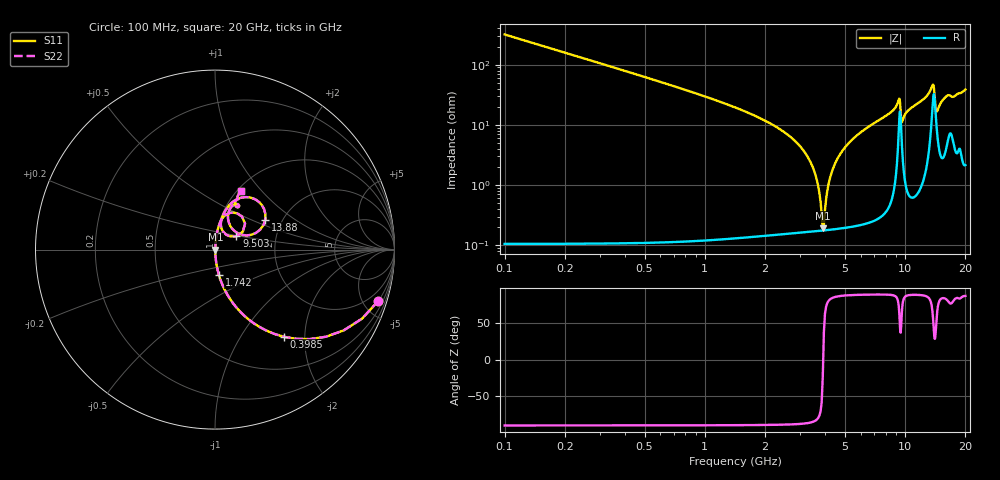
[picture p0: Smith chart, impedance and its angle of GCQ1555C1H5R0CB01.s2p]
!Murata Part Number: GCQ1555C1H5R0CB01
!These Parameters are Measured in Series Mode Connection
!Data Generated on Jan 08, 2026
!  o--ll--o
!Port1  Port2
!  o------o
!Operation Temp=25[degC], DC Bias Voltage=0[V]
!Freq. Start=100[MHz] Stop=20[GHz] 401[Steps]
# Hz S RI R 50
!Freq.(Hz) S11(Real) S11(Imag) S21(Real) S21(Imag) S12(Real) S12(Imag) S22(Real) S22(Imag)
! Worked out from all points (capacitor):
!   401 points, 100 MHz to 20 GHz, reference 50 ohm
!   read as one part in series: C = 5 pF near 199.5 MHz
!   lowest |Z| = 190 mohm at 3.881 GHz (marker M1)
!   series resonance near 3.898 GHz, so ESL is about 330 pH
!   S11 on the Smith chart (normalised r, x): 100 MHz: 1.00, -6.36; 398.5 MHz: 1.00, -1.58; 1.742 GHz: 1.00, -0.29; 9.503 GHz: 1.25, +0.19; 13.88 GHz: 1.64, +0.61; 20 GHz: 1.04, +0.77
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1e8  0.91 -0.286  0.09 0.286  0.09 0.286  0.91 -0.286
3.985e8  0.3847 -0.4858  0.6153 0.4858  0.6153 0.4858  0.3847 -0.4858
8.4625e8  0.1146 -0.317  0.8854 0.317  0.8854 0.317  0.1146 -0.317
1.74175e9  0.0223 -0.1429  0.9777 0.1429  0.9777 0.1429  0.0223 -0.1429
2.83625e9  0.00438 -0.0527  0.9956 0.0527  0.9956 0.0527  0.00438 -0.0527
3.43325e9  0.00212 -0.0209  0.9979 0.0209  0.9979 0.0209  0.00212 -0.0209
3.63225e9  0.00185 -0.0116  0.9982 0.0116  0.9982 0.0116  0.00185 -0.0116
3.881e9  0.00175 -0.000732  0.9982 0.000732  0.9982 0.000732  0.00175 -0.000732
3.9805e9  0.00178 0.00343  0.9982 -0.00343  0.9982 -0.00343  0.00178 0.00343
4.22925e9  0.00199 0.0134  0.998 -0.0134  0.998 -0.0134  0.00199 0.0134
4.677e9  0.0028 0.0303  0.9972 -0.0303  0.9972 -0.0303  0.0028 0.0303
5.473e9  0.00536 0.0575  0.9946 -0.0575  0.9946 -0.0575  0.00536 0.0575
6.7665e9  0.0122 0.098  0.9878 -0.098  0.9878 -0.098  0.0122 0.098
9.30375e9  0.1238 0.202  0.8762 -0.202  0.8762 -0.202  0.1238 0.202
9.50275e9  0.1192 0.074  0.8808 -0.074  0.8808 -0.074  0.1192 0.074
9.652e9  0.0499 0.0942  0.9501 -0.0942  0.9501 -0.0942  0.0499 0.0942
1.005e10  0.0326 0.1476  0.9674 -0.1476  0.9674 -0.1476  0.0326 0.1476
1.338325e10  0.1635 0.292  0.8365 -0.292  0.8365 -0.292  0.1635 0.292
1.388075e10  0.2801 0.1673  0.7199 -0.1673  0.7199 -0.1673  0.2801 0.1673
1.43285e10  0.1057 0.1064  0.8943 -0.1064  0.8943 -0.1064  0.1057 0.1064
1.67165e10  0.1345 0.2432  0.8655 -0.2432  0.8655 -0.2432  0.1345 0.2432
2e10  0.1434 0.3237  0.8566 -0.3237  0.8566 -0.3237  0.1434 0.3237
